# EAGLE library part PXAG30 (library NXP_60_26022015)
XA 16-bit microcontroller family The Philips Semiconductors XA (eXtended Architecture) family of 16-bit single-chip microcontrollers is powerful enough to easily handle the requirements of high performance embedded applications, yet inexpensive enough to compete in the market for high-volume, low-cost applications. The XA family provides an upward compatibility path for 80C51 users who need higher performance and 64k or more of program memory. Existing 80C51 code can also easily be translated to run on XA microcontrollers. The performance of the XA architecture supports the comprehensive bit-oriented operations of the 80C51 while incorporating support for multi-tasking operating systems and high-level languages such as C. The speed of the XA architecture, at 10 to 100 times that of the 80C51, gives designers an easy path to truly high performance embedded control. AAL Eindhoven MK
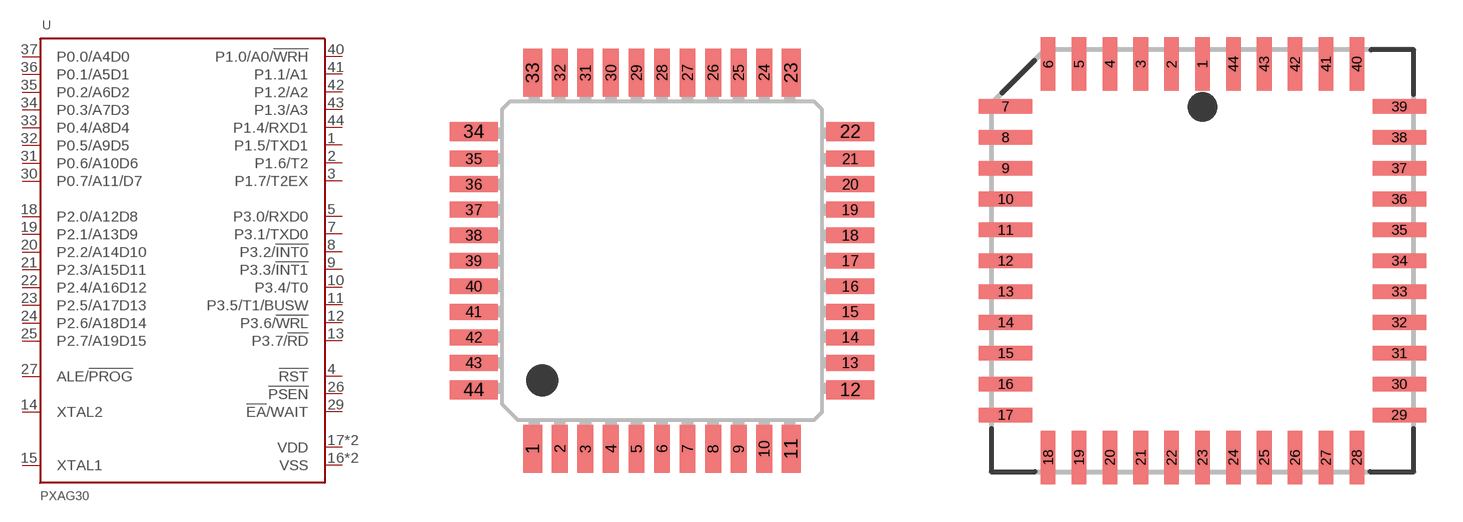
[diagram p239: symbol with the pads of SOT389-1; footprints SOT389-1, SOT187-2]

Designator prefix U

## PXAG30KBBD  [SOT389-1]
1  P1.5/TXD1
2  P1.6/T2
3  P1.7/T2EX
4  !RST!  in
5  P3.0/RXD0
7  P3.1/TXD0
8  P3.2/!INT0!
9  P3.3/!INT1!
10  P3.4/T0
11  P3.5/T1/BUSW
12  P3.6/!WRL!
13  P3.7/!RD!
14  XTAL2  out
15  XTAL1  in
16  VSS
17  VDD  pwr
18  P2.0/A12D8
19  P2.1/A13D9
20  P2.2/A14D10
21  P2.3/A15D11
22  P2.4/A16D12
23  P2.5/A17D13
24  P2.6/A18D14
25  P2.7/A19D15
26  !PSEN!  out
27  ALE/!PROG!
29  !EA!/WAIT
30  P0.7/A11/D7
31  P0.6/A10D6
32  P0.5/A9D5
33  P0.4/A8D4
34  P0.3/A7D3
35  P0.2/A6D2
36  P0.1/A5D1
37  P0.0/A4D0
38  VDD  pwr
39  VSS
40  P1.0/A0/!WRH!
41  P1.1/A1
42  P1.2/A2
43  P1.3/A3
44  P1.4/RXD1

## PXAG30KBA  [SOT187-2]
1  VSS
2  P1.0/A0/!WRH!
3  P1.1/A1
4  P1.2/A2
5  P1.3/A3
6  P1.4/RXD1
7  P1.5/TXD1
8  P1.6/T2
9  P1.7/T2EX
10  !RST!  in
11  P3.0/RXD0
13  P3.1/TXD0
14  P3.2/!INT0!
15  P3.3/!INT1!
16  P3.4/T0
17  P3.5/T1/BUSW
18  P3.6/!WRL!
19  P3.7/!RD!
20  XTAL2  out
21  XTAL1  in
22  VSS
23  VDD  pwr
24  P2.0/A12D8
25  P2.1/A13D9
26  P2.2/A14D10
27  P2.3/A15D11
28  P2.4/A16D12
29  P2.5/A17D13
30  P2.6/A18D14
31  P2.7/A19D15
32  !PSEN!  out
33  ALE/!PROG!
35  !EA!/WAIT
36  P0.7/A11/D7
37  P0.6/A10D6
38  P0.5/A9D5
39  P0.4/A8D4
40  P0.3/A7D3
41  P0.2/A6D2
42  P0.1/A5D1
43  P0.0/A4D0
44  VDD  pwr

## PXAG30KFBD  [SOT389-1]
Pads as for SOT389-1

## PXAG30KFA  [SOT187-2]
Pads as for SOT187-2

## Footprint SOT389-1 (pad centres in mm)
SOT389-1 LQFP44: plastic low profile quad flat package; 44 leads; body 10 x 10 x 1.4 mm JEDEC: MS-026 IEC: 136E08 JEITA: --
smd 0.6 x 1.5: 1 -4.05,-5.9; 11 4.05,-5.9; 23 4.05,5.9; 33 -4.05,5.9
smd 0.5 x 1.5: 2 -3.2,-5.9; 3 -2.4,-5.9; 4 -1.6,-5.9; 5 -0.8,-5.9; 6 0,-5.9; 7 0.8,-5.9; 8 1.6,-5.9; 9 2.4,-5.9; 10 3.2,-5.9; 24 3.2,5.9; 25 2.4,5.9; 26 1.6,5.9; 27 0.8,5.9; 28 0,5.9; 29 -0.8,5.9; 30 -1.6,5.9; 31 -2.4,5.9; 32 -3.2,5.9
smd 1.5 x 0.6: 12 5.9,-4.05; 22 5.9,4.05; 34 -5.9,4.05; 44 -5.9,-4.05
smd 1.5 x 0.5: 13 5.9,-3.2; 14 5.9,-2.4; 15 5.9,-1.6; 16 5.9,-0.8; 17 5.9,0; 18 5.9,0.8; 19 5.9,1.6; 20 5.9,2.4; 21 5.9,3.2; 35 -5.9,3.2; 36 -5.9,2.4; 37 -5.9,1.6; 38 -5.9,0.8; 39 -5.9,0; 40 -5.9,-0.8; 41 -5.9,-1.6; 42 -5.9,-2.4; 43 -5.9,-3.2

## Footprint SOT187-2 (pad centres in mm)
SOT187-2 PLCC44: plastic leaded chip carrier; 44 leads JEDEC: MS-018 IEC: 112E10 JEITA: EDR-7319
smd 0.6 x 2.2: 1 0,8.1; 2 -1.27,8.1; 3 -2.54,8.1; 4 -3.81,8.1; 5 -5.08,8.1; 6 -6.35,8.1; 18 -6.35,-8.1; 19 -5.08,-8.1; 20 -3.81,-8.1; 21 -2.54,-8.1; 22 -1.27,-8.1; 23 0,-8.1; 24 1.27,-8.1; 25 2.54,-8.1; 26 3.81,-8.1; 27 5.08,-8.1; 28 6.35,-8.1; 40 6.35,8.1; 41 5.08,8.1; 42 3.81,8.1; 43 2.54,8.1; 44 1.27,8.1
smd 2.2 x 0.6: 7 -8.1,6.35; 8 -8.1,5.08; 9 -8.1,3.81; 10 -8.1,2.54; 11 -8.1,1.27; 12 -8.1,0; 13 -8.1,-1.27; 14 -8.1,-2.54; 15 -8.1,-3.81; 16 -8.1,-5.08; 17 -8.1,-6.35; 29 8.1,-6.35; 30 8.1,-5.08; 31 8.1,-3.81; 32 8.1,-2.54; 33 8.1,-1.27; 34 8.1,0; 35 8.1,1.27; 36 8.1,2.54; 37 8.1,3.81; 38 8.1,5.08; 39 8.1,6.35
